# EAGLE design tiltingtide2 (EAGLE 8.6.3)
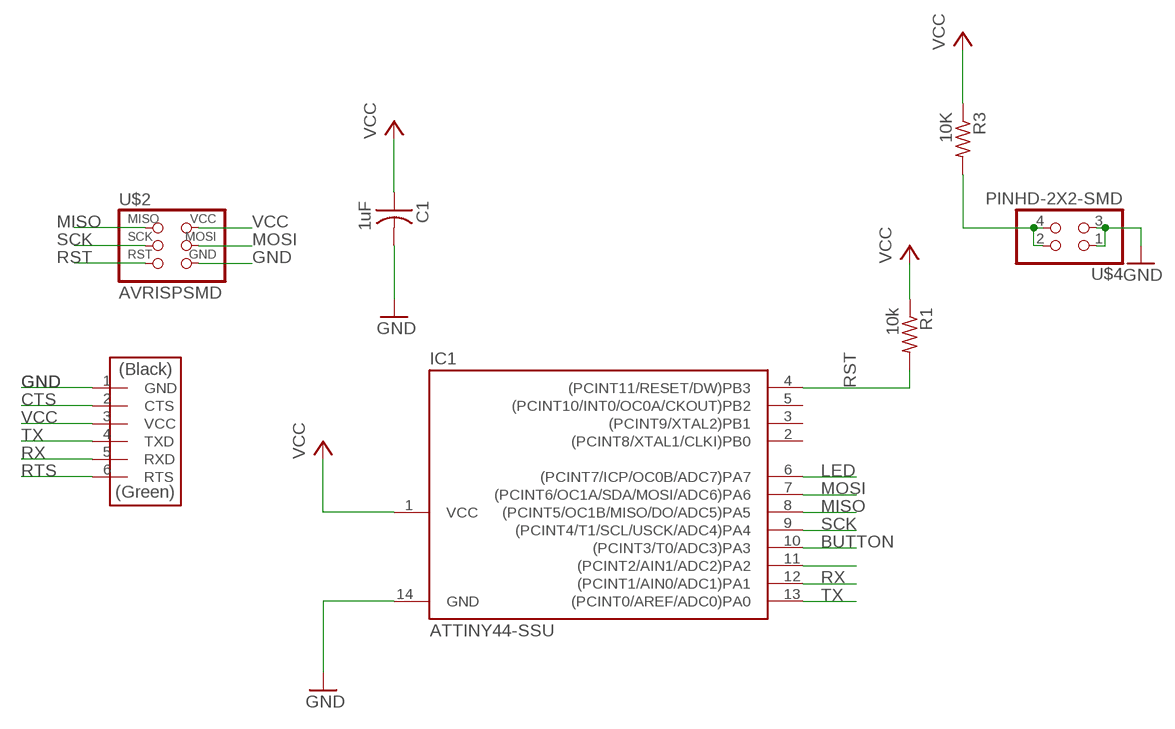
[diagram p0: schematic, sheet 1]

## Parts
C1  1uF  CAP-US1206  [C1206]
IC1  ATTINY44-SSU  [SOIC14]
R1  10k  RES-US1206  [R1206]
R3  10K  RES-US1206  [R1206]
U$2  AVRISPSMD  [2X03SMD]
U$3  FTDI-SMD-HEADER  [1X06SMD]
U$4  PINHD-2X2-SMD  [2X02SMD]

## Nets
BUTTON: IC1.10((PCINT3/T0/ADC3)PA3) R3.2 U$4.2 U$4.4
CTS: U$3.2(CTS)
GND: C1.2 IC1.14(GND) U$2.6(GND) U$3.1(GND) U$4.1 U$4.3
LED: IC1.6((PCINT7/ICP/OC0B/ADC7)PA7)
MISO: IC1.8((PCINT5/OC1B/MISO/DO/ADC5)PA5) U$2.1(MISO)
MOSI: IC1.7((PCINT6/OC1A/SDA/MOSI/ADC6)PA6) U$2.4(MOSI)
N$24: IC1.11((PCINT2/AIN1/ADC2)PA2)
RST: IC1.4((PCINT11/RESET/DW)PB3) R1.2 U$2.5(RST)
RTS: U$3.6(RTS)
RX: IC1.12((PCINT1/AIN0/ADC1)PA1) U$3.5(RXD)
SCK: IC1.9((PCINT4/T1/SCL/USCK/ADC4)PA4) U$2.3(SCK)
TX: IC1.13((PCINT0/AREF/ADC0)PA0) U$3.4(TXD)
VCC: C1.1 IC1.1(VCC) R1.1 R3.1 U$2.2(VCC) U$3.3(VCC)
Unconnected: IC1.2((PCINT8/XTAL1/CLKI)PB0) IC1.3((PCINT9/XTAL2)PB1) IC1.5((PCINT10/INT0/OC0A/CKOUT)PB2)

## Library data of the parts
C1 = fab:CAP-US
IC1 = fab:ATTINY44
R1 R3 = fab:RES-US: Resistor (US Symbol)
U$2 = fab:AVRISP
U$3 = fab:FTDI-SMD-HEADER
U$4 = fab:PINHD-2X2-SMD

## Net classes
0 default: width 0.03 mm, drill 0.051 mm, clearance 0.025 mm

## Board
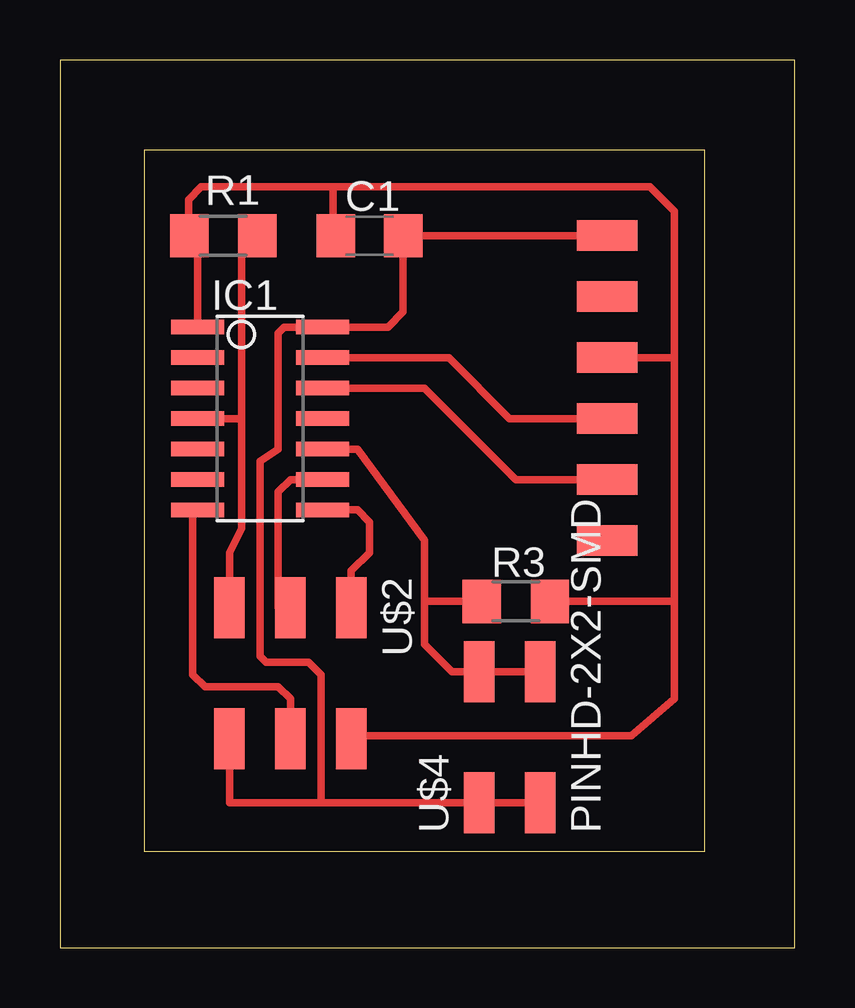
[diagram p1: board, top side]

Size 30.64 x 36.99 mm. Coordinates in mm from the lower left corner, seen from the top.
Outline: 0,0 30.64,0 30.64,36.99 0,36.99 0,0
Copper layers (1*16): Top 0.035mm / dielectric 1.5mm / Bottom 0.035mm
Design rules "default *": minimum track width 0.75mil, minimum drill 0.35mm, track to track 6mil, track to pad 6mil, pad to pad 6mil, via to via 6mil, smd to smd 6mil, copper to edge 40mil, drill to drill 6mil, minimum pad ring 10mil, minimum via ring 8mil, stop-mask expansion 4mil, vias tented up to drill 0mil, thermal gap 10mil
Milling: area 3.5,4 to 26.9,33.2

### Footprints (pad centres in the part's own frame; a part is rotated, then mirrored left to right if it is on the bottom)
C1206 = smd 1.6 x 1.8: 1 -1.4,0; 2 1.4,0
SOIC14 = smd 0.61 x 2.21: 1 -3.81,-2.603; 2 -2.54,-2.603; 3 -1.27,-2.603; 4 0,-2.603; 5 1.27,-2.603; 6 2.54,-2.603; 7 3.81,-2.603; 8 3.81,2.603; 9 2.54,2.603; 10 1.27,2.603; 11 0,2.603; 12 -1.27,2.603; 13 -2.54,2.603; 14 -3.81,2.603
R1206 = smd 1.6 x 1.803: 1 -1.422,0; 2 1.422,0
2X03SMD = smd 2.54 x 1.27: 1 -2.54,2.54; 2 2.92,2.54; 3 -2.54,0; 4 2.92,0; 5 -2.54,-2.54; 6 2.92,-2.54
1X06SMD = smd 2.54 x 1.27: 1 0,6.35; 2 0,3.81; 3 0,1.27; 4 0,-1.27; 5 0,-3.81; 6 0,-6.35
2X02SMD = smd 2.54 x 1.27: 1 -2.54,1.27; 2 2.92,1.27; 3 -2.54,-1.27; 4 2.92,-1.27

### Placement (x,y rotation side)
C1  12.91,29.67 0 top
IC1  8.34,22.05 270 top
R1  6.81,29.67 0 top
R3  19,14.43 180 top
U$2  9.61,11.64 270 top
U$3  22.81,23.32 0 top
U$4  18.75,8.59 90 top

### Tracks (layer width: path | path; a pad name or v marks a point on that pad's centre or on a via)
BUTTON
  Top 0.305: IC1.10 12.4,20.78 15.19,16.97 15.19,14.43 | R3.2 15.19,14.43 | 15.19,14.43 15.19,12.65 16.34,11.51 U$4.2 U$4.4
GND
  Top 0.152: C1.2
  Top 0.305: 10.88,6.05 10.37,6.05 7.07,6.05 U$2.6 | U$3.1 C1.2 14.3,26.5 13.67,25.86 IC1.14 9.35,25.86 9.1,25.61 9.1,20.78 8.34,20.27 8.34,12.15 8.59,11.89 10.37,11.89 10.88,11.38 10.88,6.05 | U$4.3 U$4.1 10.88,6.05
MISO
  Top 0.305: U$2.1 12.15,15.7 12.91,16.46 12.91,17.73 12.4,18.24 IC1.8
MOSI
  Top 0.152: 5.8,18.24 IC1.7
  Top 0.305: U$2.4 9.61,10.37 9.1,10.88 6.05,10.88 5.54,11.38 5.54,18.05 IC1.7
RST
  Top 0.152: 7.57,29.27 R1.2
  Top 0.305: U$2.5 7.07,16.46 7.57,17.48 7.57,22.05 | 7.57,22.05 7.57,29.27 | IC1.4 7.57,22.05
RX
  Top 0.305: IC1.12 15.19,23.32 19,19.51 U$3.5
SCK
  Top 0.152: U$2.3 9.1,14.18
  Top 0.305: 9.1,14.18 9.1,19 9.61,19.51 IC1.9
TX
  Top 0.305: IC1.13 16.21,24.59 18.75,22.05 U$3.4
VCC
  Top 0.152: 5.73,29.67 5.54,29.67 R1.1 | 12.27,8.84 U$2.2
  Top 0.305: 25.61,14.43 25.61,10.37 23.83,8.84 12.27,8.84 | 25.61,14.43 25.61,24.59 | 25.61,24.59 U$3.3 | 25.61,24.59 25.61,30.69 24.59,31.7 11.38,31.7 | R1.1 5.36,29.7 5.36,31.17 5.89,31.7 11.38,31.7 | 11.38,31.7 11.38,29.8 C1.1 | 25.61,14.43 R3.1 | IC1.1 5.73,29.48 5.54,29.67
